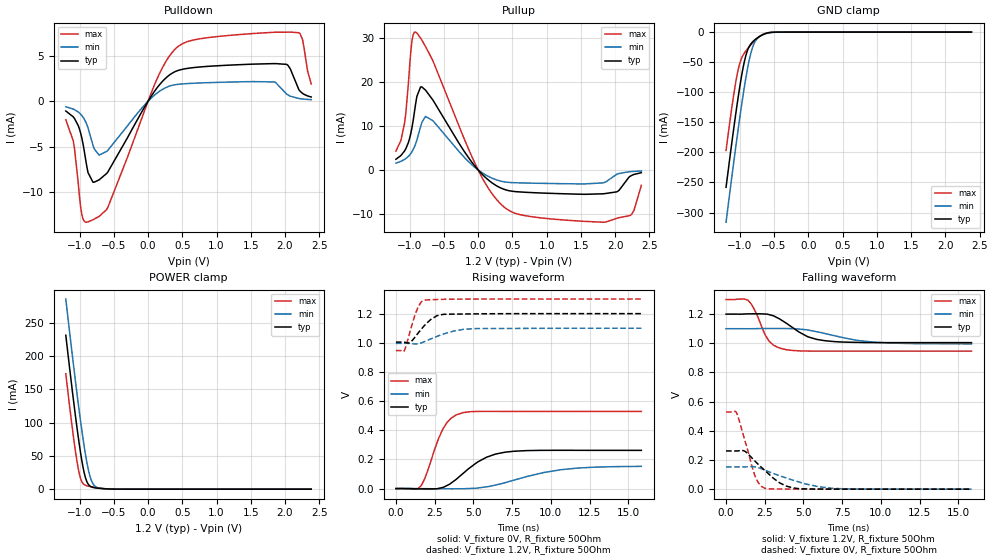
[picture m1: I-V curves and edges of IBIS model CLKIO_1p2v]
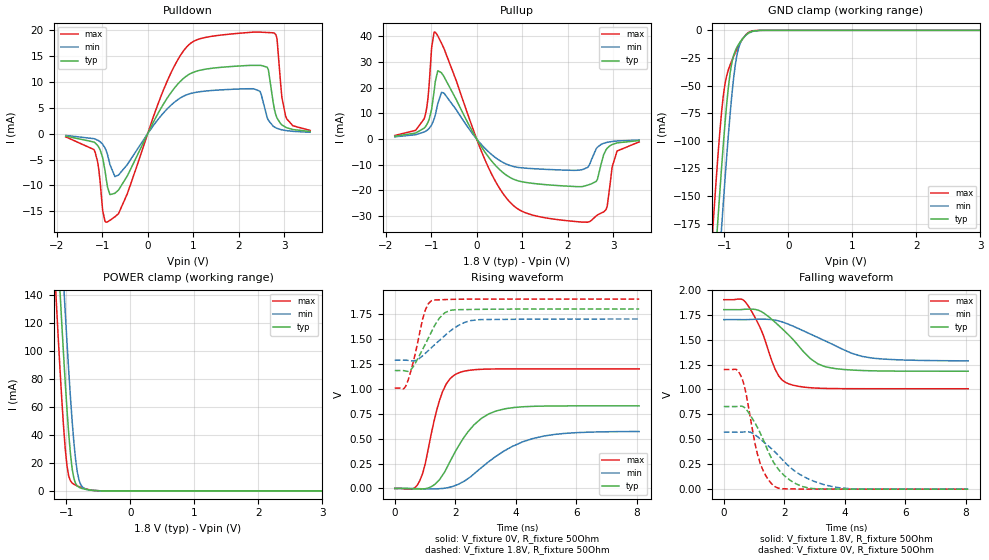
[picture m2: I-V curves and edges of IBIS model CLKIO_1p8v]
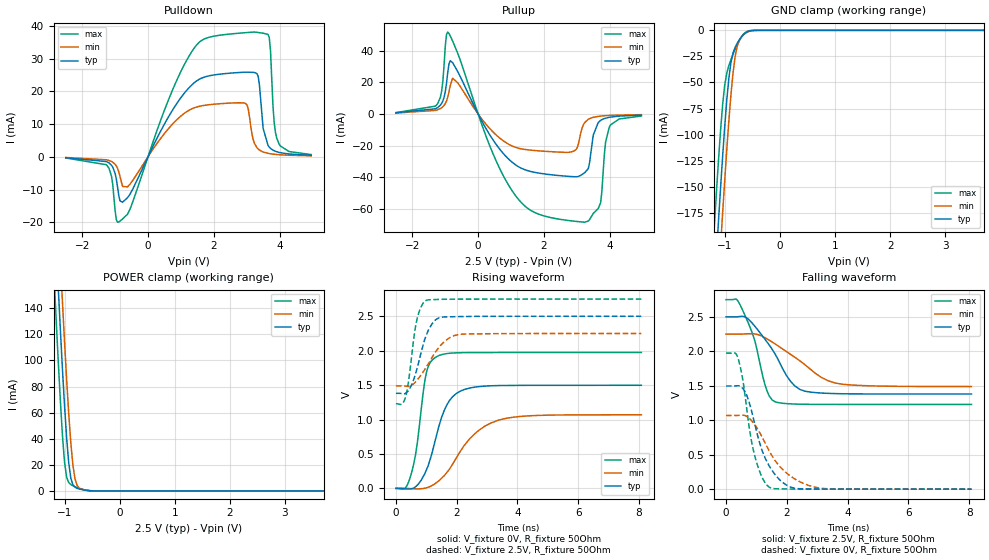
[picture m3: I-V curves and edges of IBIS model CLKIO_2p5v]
|Texas Instruments Incorporated
|Low power Stereo ADC with Embeded miniDSP
|for Wireless Handsets and Portable Audio
| Marketing part#   Voltage Range(Digital)   Package-type   #pin
|TLV320ADC3101IRGER   1.2V to 3.3V   VQFN   24
|TLV320ADC3101IRGET   1.2V to 3.3V   VQFN   24
[IBIS Ver]   4.0
[File name]   tlv320adc3101.ibs
[File Rev]   1.0
[Date]   06/13/2011
[Source]   Texas Instruments Incorporated.
   Analog-eLab, HPA
   12500 TI Blvd
   Dallas, TX -75243
   For Support e-mail: elab_ibis@list.ti.com
[Notes]   Revision History:
   1.0: 06/13/2011
   - Initial version of the model
   - Initial Model generated from simulations.
   - Model not matched to measurements
   - ccomp values are based on PVT conditions although listed
   in numerical order.
   - CLK_IO model is split into 4 models (CLKIO_1p2v, CLKIO_1p8v
   CLKIO_2p5v, CLKIO_3p3v) based operating voltages (1.2V, 1.8V,
   2.5V and 3.3V).
   - DATA model is split into 4 models (DATA_1p2v, DATA_1p8v
   DATA_2p5v, DATA_3p3v) based operating voltages (1.2V, 1.8V,
   2.5V and 3.3V).
   - INPUT model is split into 4 models (INPUT_1p2v, INPUT_1p8v
   INPUT_2p5v, INPUT_3p3v) based operating voltages (1.2V, 1.8V,
   2.5V and 3.3V).
   - I2C_IO model is split into 4 models (SDA_1p2v, SDA_1p8v
   SDA_2p5v, SDA_3p3v) based operating voltages (1.2V, 1.8V,
   2.5V and 3.3V).
   - Non-monotonicity warnings on DATA and CLK_IO buffer are
   reflection of spice simulations and can be ignored.
[Disclaimer]
 This product is designed as an aid for customers of Texas Instruments.
 No warranties, either expressed or implied, with respect to this third
 party software (if any) or with respect to its fitness for any
 particular purpose is claimed by Texas Instruments or the author. The
 software (if any) is provided solely on an "as is" basis. The entire
 risk as to its quality and performance is with the customer
[Copyright] (C) Copyright 2011 Texas Instruments Incorporated.
   All rights reserved.
|   TLV320ADC3101
[Component]   tlv320adc3101
[Manufacturer] TI
[Package]   | 24 pin  package
| variable   typ   min   max
R_pkg   0.0746   0.0381   0.0838
L_pkg   1.09nH   0.81nH   1.21nH
C_pkg   0.148pF   0.126pF   0.195pF
|-------------------------PIN------------------------------------------------
[Pin] signal_name  model_name  R_pin  L_pin C_pin
1   BCLK   CLK_IO   0.07924   1.11525nH   0.12716pF
2   WCLK   CLK_IO   0.07327   1.05316nH   0.1487pF
3   DOUT   DATA   0.07354   1.05587nH   0.14822pF
4   RESETB   INPUT   0.07981   1.14793nH   0.1523pF
5   MICBIAS1   TERM   0.07489   1.07511nH   0.14724pF
6   IN3L   TERM   0.07839   1.12703nH   0.15083pF
7   IN2L   TERM   0.08148   1.17211nH   0.15382pF
8   IN1L   TERM   0.07748   1.11307nH   0.15103pF
9   AVSS   GND   0.03814   0.80558nH   0.15549pF
10   AVDD   POWER   0.07565   1.08748nH   0.12622pF
11   IN1R   TERM   0.07727   1.10694nH   0.15pF
12   IN2R   TERM   0.08077   1.1574nH   0.15299pF
13   IN3R   TERM   0.07839   1.11986nH   0.15072pF
14   MICBIAS2   TERM   0.07489   1.06758nH   0.14704pF
15   I2C_ADR0   INPUT   0.07998   1.14372nH   0.15228pF
16   I2C_ADR1   INPUT   0.07361   1.04912nH   0.14805pF
17   SCL   I2C_IO   0.07322   1.04451nH   0.14849pF
18   SDA   I2C_IO   0.07924   1.13822nH   0.12709pF
19   DMDIN_GPIO1   CLK_IO   0.08359   1.20475nH   0.13135pF
20   DMCLK_GPIO2   CLK_IO   0.07633   1.09324nH   0.1509pF
21   IVODD   POWER   0.07496   1.07238nH   0.15063pF
22   DVDD   POWER   0.07812   1.12112nH   0.15804pF
23   DVSS   GND   0.04448   0.97782nH   0.19585pF
24   MCLK   INPUT   0.08381   1.20712nH   0.15521pF
[Model Selector] CLK_IO
CLKIO_3p3v  3.3V cmos I/O
CLKIO_2p5v  2.5V cmos I/O
CLKIO_1p8v  1.8V cmos I/O
CLKIO_1p2v  1.2V cmos I/O
[Model Selector] DATA
DATA_3p3v   3.3V tristate output
DATA_2p5v   2.5V tristate output
DATA_1p8v   1.8V tristate output
DATA_1p2v   1.2V tristate output
[Model Selector] INPUT
INPUT_3p3v  3.3V cmos input
INPUT_2p5v  2.5V cmos input
INPUT_1p8v  1.8V cmos input
INPUT_1p2v  1.2V cmos input
[Model Selector] I2C_IO
SDA_3p3v  3.3V open I/O
SDA_2p5v  2.5V open I/O
SDA_1p8v  1.8V open I/O
SDA_1p2v  1.2V open I/O
[Model]  TERM
Model_type Terminator
C_comp   0   0   0
[Voltage Range]  3.3  3.0  3.6
[Temperature Range] 27   85   -40
| Models and submodels in the file (17): CLKIO_1p2v (I/O), CLKIO_1p8v (I/O), CLKIO_2p5v (I/O), CLKIO_3p3v (I/O), DATA_1p2v (3-state), DATA_1p8v (3-state), DATA_2p5v (3-state), DATA_3p3v (3-state), INPUT_1p2v (Input), INPUT_1p8v (Input), INPUT_2p5v (Input), INPUT_3p3v (Input), SDA_1p2v (I/O_open_drain), SDA_1p8v (I/O_open_drain), SDA_2p5v (I/O_open_drain), SDA_3p3v (I/O_open_drain), TERM (Terminator)
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|   CLKIO_1p2v
[Model]   CLKIO_1p2v
Model_type   I/O
Polarity   Non-Inverting
Enable   Active-High
Vinl = 0.36
Vinh = 0.84
Vmeas = 0.6
Vref = 0
Cref = 5pF
Rref = 1000000
|   typ   min   max
C_comp   1.630pF   1.592pF   1.693pF
[Voltage Range]   1.2   1.1   1.3
[Temperature Range]   27   85   -40
[Pullup Reference]   1.2   1.1   1.3
[Pulldown Reference]   -0   -0   -0
[Power Clamp Reference]   1.2   1.1   1.3
[GND Clamp Reference]   -0   -0   -0
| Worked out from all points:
|   slope of the pulldown table from 0 to 0.18 V, typ, clamps not added: 93.3 ohm
|   slope of the pullup table from 0 to 0.18 V, typ, clamps not added: 67.6 ohm
|   GND clamp passes 1 mA (typ) near -0.57 V on its own axis
|   POWER clamp passes 1 mA (typ) near -0.68 V on its own axis
|   falling waveform, V_fixture 1.2V, R_fixture 50Ohm: 20-80 % time 1.76ns typ, 2.87ns min, 919ps max; typ from 1.2 V to 1 V
|   rising waveform, V_fixture 0V, R_fixture 50Ohm: 20-80 % time 2ns typ, 3.54ns min, 1.13ns max; typ from 0 V to 0.262 V
|   rising waveform, V_fixture 1.2V, R_fixture 50Ohm: 20-80 % time 996ps typ, 1.64ns min, 610ps max; typ from 1 V to 1.2 V
|   falling waveform, V_fixture 0V, R_fixture 50Ohm: 20-80 % time 1.64ns typ, 2.66ns min, 845ps max; typ from 0.262 V to 0 V
[Pulldown]
|   Voltage   I(typ)   I(min)   I(max)
-1.2V     -1.07mA    -597.3uA   -2.042mA
-1.092V   -1.709mA   -856.2uA   -4.33mA
-1.02V    -2.651mA   -1.171mA   -8.868mA
-966mV    -4.044mA   -1.567mA   -12.48mA
-894mV    -7.151mA   -2.544mA   -13.31mA
-714mV    -8.651mA   -5.923mA   -12.68mA
-588mV    -7.806mA   -5.41mA    -11.71mA
168mV     1.822mA    1.102mA    3.055mA
492mV     3.504mA    1.906mA    6.299mA
2.022V    4.065mA    805.4uA    7.611mA
2.202V    1.268mA    305.9uA    7.546mA
2.382V    470.8uA    178.6uA    1.904mA
[GND Clamp]
|   Voltage   I(typ)   I(min)   I(max)
-1.2V     -258.1mA   -316.1mA   -196.8mA
-1.11V    -179mA     -235.8mA   -121mA
-1.038V   -119.8mA   -174mA     -70.54mA
-984mV    -79.98mA   -130mA     -46.43mA
-930mV    -47.68mA   -89.38mA   -34.41mA
-876mV    -27.29mA   -54.35mA   -26.35mA
-822mV    -17.42mA   -28.48mA   -19.29mA
-768mV    -11.74mA   -14.04mA   -12.97mA
-714mV    -7.456mA   -7.504mA   -7.628mA
-624mV    -2.511mA   -2.629mA   -1.885mA
-534mV    -448.7uA   -620uA     -192.6uA
2.382V    0A         0A         0A
[Pullup]
|   Voltage   I(typ)   I(min)   I(max)
-1.2V     2.421mA    1.547mA    4.272mA
-1.074V   4.296mA    2.378mA    10.6mA
-966mV    9.578mA    4.11mA     29.26mA
-912mV    15.02mA    5.927mA    31.26mA
-840mV    18.83mA    9.821mA    29.89mA
-768mV    18.09mA    12.13mA    27.99mA
6mV       -105.3uA   -68.85uA   -187.8uA
420mV     -4.595mA   -2.784mA   -8.894mA
1.86V     -5.348mA   -2.744mA   -11.81mA
2.04V     -4.823mA   -895.3uA   -10.89mA
2.238V    -1.262mA   -368.8uA   -10.11mA
2.382V    -626.9uA   -250.3uA   -3.496mA
[POWER Clamp]
|   Voltage   I(typ)   I(min)   I(max)
-1.2V     231.1mA    285.3mA    173.2mA
-1.128V   167.6mA    221.3mA    110.7mA
-1.074V   122.1mA    174.7mA    67.66mA
-1.038V   93.31mA    144.7mA    42.54mA
-1.002V   66.55mA    115.7mA    22.83mA
-948mV    32.67mA    75.35mA    8.401mA
-894mV    11.57mA    41.03mA    5.093mA
-840mV    4.122mA    16.94mA    3.804mA
-804mV    2.641mA    8.113mA    3.132mA
-768mV    1.932mA    3.889mA    2.523mA
-480mV    49.56uA    80.74uA    34.71uA
2.382V    0A         0A         0A
[Ramp]
R_load = 50
|   typ   min   max
dV/dt_r   0.157257/2.00205e-009 0.0913656/3.53688e-009  0.317475/1.12719e-009
dV/dt_f   0.117245/1.76151e-009  0.062354/2.86788e-009  0.212217/9.19327e-010
[Falling Waveform]
V_fixture = 1.2V
V_fixture_min = 1.1V
V_fixture_max = 1.3V
R_fixture = 50Ohm
C_fixture = 0F
|   Time   V(typ)   V(min)   V(max)
0s        1.2V       1.1V       1.3V
1.423ns   1.202V     1.1V       1.295V
1.857ns   1.202V     1.1V       1.226V
2.507ns   1.201V     1.101V     1.061V
2.772ns   1.197V     1.101V     1.015V
3.906ns   1.136V     1.101V     955.9mV
5.271ns   1.045V     1.091V     946.7mV
6.438ns   1.017V     1.066V     946.2mV
9.582ns   1.005V     1.007V     946.3mV
15.84ns   1.005V     996.1mV    946.3mV
[Rising Waveform]
V_fixture = 0V
V_fixture_min = 0V
V_fixture_max = 0V
R_fixture = 50Ohm
C_fixture = 0F
|   Time   V(typ)   V(min)   V(max)
0s        -1.318uV   -3.119uV   -2.104uV
1.207ns   -1.529mV   132.3uV    -4.123mV
1.64ns    -2.22mV    -319uV     21.2mV
3.037ns   7.794mV    -1.349mV   409.6mV
3.567ns   37.87mV    -1.431mV   483.3mV
4.362ns   106.2mV    -1.186mV   521.5mV
5.855ns   215.3mV    12mV       529.7mV
7.021ns   249.2mV    39.65mV    529.4mV
10.66ns   262.5mV    129.4mV    529.1mV
15.84ns   262.1mV    152.3mV    529.1mV
[Rising Waveform]
V_fixture = 1.2V
V_fixture_min = 1.1V
V_fixture_max = 1.3V
R_fixture = 50Ohm
C_fixture = 0F
|   Time   V(typ)   V(min)   V(max)
0s        1.005V     996.1mV    946.3mV
533.2ps   1.004V     996.5mV    945.1mV
942ps     1.005V     995mV      1.088V
1.423ns   1.065V     993.2mV    1.245V
1.64ns    1.094V     999.4mV    1.282V
1.857ns   1.12V      1.008V     1.293V
2.653ns   1.186V     1.044V     1.297V
3.06ns    1.195V     1.06V      1.298V
5.179ns   1.198V     1.098V     1.3V
15.84ns   1.2V       1.1V       1.3V
[Falling Waveform]
|Gnd
V_fixture = 0V
V_fixture_min = 0V
V_fixture_max = 0V
R_fixture = 50Ohm
C_fixture = 0F
|   Time   V(typ)   V(min)   V(max)
0s        262.1mV    152.5mV    529.1mV
682.4ps   262mV      152.3mV    522.6mV
1.169ns   262.3mV    152.6mV    351.2mV
1.857ns   193.5mV    153mV      93.19mV
2.074ns   170.8mV    147.7mV    45.25mV
2.507ns   128.1mV    130.5mV    5.84mV
3.467ns   42.82mV    91.7mV     1.137mV
4.688ns   3.395mV    49.91mV    156.3uV
7.671ns   291.7uV    1.874mV    2.37uV
15.84ns   -1.062uV   18.06uV    128.5nV
|   CLKIO_1p8v
[Model]   CLKIO_1p8v
Model_type   I/O
Polarity   Non-Inverting
Enable   Active-High
Vinl = 0.54
Vinh = 1.26
Vmeas = 0.9
Vref = 0
Cref = 5pF
Rref = 1000000
|   typ   min   max
C_comp   1.630pF   1.592pF   1.693pF
[Voltage Range]   1.8   1.7   1.9
[Temperature Range]   27   85   -40
[Pullup Reference]   1.8   1.7   1.9
[Pulldown Reference]   -0   -0   -0
[Power Clamp Reference]   1.8   1.7   1.9
[GND Clamp Reference]   -0   -0   -0
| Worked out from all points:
|   slope of the pulldown table from 0 to 0.27 V, typ, clamps not added: 59 ohm
|   slope of the pullup table from 0 to 0.27 V, typ, clamps not added: 37.3 ohm
|   GND clamp passes 1 mA (typ) near -0.57 V on its own axis
|   POWER clamp passes 1 mA (typ) near -0.68 V on its own axis
|   falling waveform, V_fixture 1.8V, R_fixture 50Ohm: 20-80 % time 1.19ns typ, 1.76ns min, 694ps max; typ from 1.8 V to 1.18 V
|   rising waveform, V_fixture 0V, R_fixture 50Ohm: 20-80 % time 1.06ns typ, 1.65ns min, 567ps max; typ from 0 V to 0.828 V
|   rising waveform, V_fixture 1.8V, R_fixture 50Ohm: 20-80 % time 639ps typ, 949ps min, 403ps max; typ from 1.18 V to 1.8 V
|   falling waveform, V_fixture 0V, R_fixture 50Ohm: 20-80 % time 870ps typ, 1.33ns min, 495ps max; typ from 0.828 V to 0 V
[Pulldown]
|   Voltage   I(typ)   I(min)   I(max)
-1.8V     -446.7uA   -316.8uA   -599.3uA
-1.179V   -1.6mA     -947.7uA   -3.058mA
-1.071V   -2.646mA   -1.378mA   -7.075mA
-990mV    -4.574mA   -2.008mA   -14.74mA
-882mV    -10.33mA   -4.037mA   -17.03mA
-639mV    -10.88mA   -7.975mA   -15.44mA
819mV     10.93mA    7.395mA    16.38mA
2.331V    13.24mA    8.707mA    19.67mA
2.655V    12.35mA    2.589mA    19.58mA
2.817V    3.697mA    1.159mA    19.19mA
3.033V    1.263mA    634.3uA    3.405mA
3.573V    443.3uA    289.3uA    650.2uA
[GND Clamp]
|   Voltage   I(typ)   I(min)   I(max)
-1.8V     -825.7mA   -883.1mA   -764.8mA
-1.179V   -239.3mA   -297.1mA   -178.4mA
-1.125V   -191.9mA   -248.9mA   -133mA
-1.098V   -168.8mA   -225.3mA   -111.7mA
-1.044V   -124.5mA   -179mA     -74.1mA
-990mV    -84.11mA   -134.8mA   -48.37mA
-936mV    -50.74mA   -93.67mA   -35.44mA
-882mV    -28.93mA   -57.86mA   -27.19mA
-828mV    -18.22mA   -30.79mA   -20.04mA
-747mV    -9.958mA   -10.88mA   -10.76mA
-612mV    -2.077mA   -2.232mA   -1.464mA
3.573V    0A         0A         0A
[Pullup]
|   Voltage   I(typ)   I(min)   I(max)
-1.8V     1.07mA     844.6uA    1.357mA
-1.152V   4.258mA    2.717mA    7.917mA
-1.071V   6.428mA    3.67mA     15.74mA
-936mV    18.47mA    7.689mA    41.63mA
-855mV    26.58mA    13.72mA    40.19mA
-720mV    24.34mA    17.91mA    35.31mA
252mV     -6.828mA   -4.846mA   -10.85mA
954mV     -16.5mA    -11.17mA   -27.75mA
2.493V    -17.65mA   -9.494mA   -32.08mA
2.844V    -4.206mA   -1.404mA   -27.53mA
3.087V    -1.515mA   -777.6uA   -4.683mA
3.573V    -628uA     -402.2uA   -1.128mA
[POWER Clamp]
|   Voltage   I(typ)   I(min)   I(max)
-1.8V     798.6mA    851.4mA    743.1mA
-1.179V   212.3mA    266.5mA    154.6mA
-1.152V   188.5mA    242.4mA    131.1mA
-1.098V   142mA      195.2mA    86.23mA
-1.044V   97.98mA    149.6mA    46.43mA
-1.017V   77.4mA     127.6mA    30.18mA
-990mV    58.24mA    106.4mA    18mA
-909mV    15.86mA    49.74mA    5.628mA
-855mV    5.278mA    22.34mA    4.111mA
-801mV    2.564mA    7.615mA    3.079mA
-450mV    23.52uA    44.09uA    13.85uA
3.573V    0A         0A         0A
[Ramp]
R_load = 50
|   typ   min   max
dV/dt_r   0.497073/1.06086e-009  0.342582/1.65226e-009  0.719771/5.67278e-010
dV/dt_f   0.370361/1.18967e-009  0.247646/1.75578e-009  0.535854/6.94284e-010
[Falling Waveform]
V_fixture = 1.8V
V_fixture_min = 1.7V
V_fixture_max = 1.9V
R_fixture = 50Ohm
C_fixture = 0F
|   Time   V(typ)   V(min)   V(max)
0s        1.8V       1.7V       1.9V
753.7ps   1.804V     1.7V       1.861V
1.204ns   1.786V     1.704V     1.618V
1.697ns   1.673V     1.695V     1.202V
1.932ns   1.607V     1.677V     1.092V
2.167ns   1.538V     1.65V      1.054V
2.859ns   1.309V     1.556V     1.017V
3.349ns   1.228V     1.487V     1.01V
4.909ns   1.187V     1.314V     1.007V
8.073ns   1.183V     1.287V     1.007V
[Rising Waveform]
V_fixture = 0V
V_fixture_min = 0V
V_fixture_max = 0V
R_fixture = 50Ohm
C_fixture = 0F
|   Time   V(typ)   V(min)   V(max)
0s        -6.278uV   -2.564uV   -11.23uV
606.8ps   -4.343mV   -81.27uV   -2.123mV
828.1ps   -5.588mV   -2.675mV   78.44mV
1.485ns   91.64mV    -2.191mV   890.4mV
1.697ns   194.1mV    5.008mV    1.046V
2.05ns    396.1mV    35.81mV    1.152V
2.859ns   702.6mV    208.3mV    1.195V
3.651ns   799.9mV    382.7mV    1.199V
5.256ns   827.4mV    541.2mV    1.199V
8.073ns   828.4mV    571mV      1.2V
[Rising Waveform]
V_fixture = 1.8V
V_fixture_min = 1.7V
V_fixture_max = 1.9V
R_fixture = 50Ohm
C_fixture = 0F
|   Time   V(typ)   V(min)   V(max)
0s        1.183V     1.286V     1.007V
289.8ps   1.182V     1.287V     1.001V
389ps     1.176V     1.286V     1.044V
606.8ps   1.222V     1.279V     1.264V
922ps     1.397V     1.332V     1.702V
1.016ns   1.452V     1.358V     1.795V
1.204ns   1.566V     1.41V      1.882V
1.648ns   1.762V     1.532V     1.895V
2.512ns   1.795V     1.684V     1.899V
8.073ns   1.8V       1.7V       1.9V
[Falling Waveform]
|Gnd
V_fixture = 0V
V_fixture_min = 0V
V_fixture_max = 0V
R_fixture = 50Ohm
C_fixture = 0F
|   Time   V(typ)   V(min)   V(max)
0s        828.4mV    571.6mV    1.2V
400ps     828.4mV    571.4mV    1.201V
557.9ps   832.5mV    571.7mV    1.14V
704.7ps   812.2mV    574.4mV    1.001V
1.016ns   671.7mV    548.8mV    478.4mV
1.204ns   562.1mV    503.7mV    258.2mV
1.697ns   246mV      370.7mV    24.38mV
2.416ns   49.46mV    167.2mV    1.866mV
3.596ns   1.62mV     24.72mV    171uV
8.073ns   1.935uV    79.25uV    -2.062uV
|   CLKIO_2p5v
[Model]   CLKIO_2p5v
Model_type   I/O
Polarity   Non-Inverting
Enable   Active-High
Vinl = 0.75
Vinh = 1.75
Vmeas = 1.25
Vref = 0
Cref = 5pF
Rref = 1000000
|   typ   min   max
C_comp   1.630pF   1.592pF   1.693pF
[Voltage Range]   2.5   2.25   2.75
[Temperature Range]   27   85   -40
[Pullup Reference]   2.5   2.25   2.75
[Pulldown Reference]   -0   -0   -0
[Power Clamp Reference]   2.5   2.25   2.75
[GND Clamp Reference]   -0   -0   -0
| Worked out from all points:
|   slope of the pulldown table from 0 to 0.375 V, typ, clamps not added: 48.9 ohm
|   slope of the pullup table from 0 to 0.375 V, typ, clamps not added: 27 ohm
|   GND clamp passes 1 mA (typ) near -0.57 V on its own axis
|   POWER clamp passes 1 mA (typ) near -0.68 V on its own axis
|   falling waveform, V_fixture 2.5V, R_fixture 50Ohm: 20-80 % time 953ps typ, 1.42ns min, 572ps max; typ from 2.5 V to 1.38 V
|   rising waveform, V_fixture 0V, R_fixture 50Ohm: 20-80 % time 628ps typ, 1.12ns min, 354ps max; typ from 0 V to 1.5 V
|   rising waveform, V_fixture 2.5V, R_fixture 50Ohm: 20-80 % time 444ps typ, 700ps min, 282ps max; typ from 1.38 V to 2.5 V
|   falling waveform, V_fixture 0V, R_fixture 50Ohm: 20-80 % time 673ps typ, 986ps min, 449ps max; typ from 1.5 V to 0 V
[Pulldown]
|   Voltage   I(typ)   I(min)   I(max)
-2.5V     -290.5uA   -214.9uA   -365.9uA
-1.262V   -1.448mA   -911.1uA   -2.421mA
-887.5mV  -11.93mA   -4.616mA   -19.88mA
-625mV    -12.51mA   -9.182mA   -17.54mA
1.4V      22.56mA    14.92mA    33.12mA
2.975V    25.83mA    16.23mA    37.89mA
3.237V    25.73mA    4.081mA    38.06mA
3.35V     24.52mA    2.367mA    37.94mA
3.688V    2.949mA    982uA      36.34mA
3.837V    1.849mA    772.8uA    10.3mA
3.987V    1.335mA    635.9uA    3.857mA
4.963V    465.7uA    292.8uA    680.3uA
[GND Clamp]
|   Voltage   I(typ)   I(min)   I(max)
-2.5V     -1.51A     -1.565A    -1.451A
-1.188V   -246.9mA   -304.8mA   -185.8mA
-1.113V   -181.2mA   -237.9mA   -123mA
-1.075V   -149.6mA   -205.4mA   -94.66mA
-1.038V   -119.4mA   -173.6mA   -70.25mA
-1V       -91.19mA   -142.8mA   -52mA
-925mV    -45.24mA   -85.86mA   -33.59mA
-887.5mV  -30.55mA   -61.18mA   -27.96mA
-812.5mV  -16.25mA   -25.13mA   -18.12mA
-775mV    -12.38mA   -15.34mA   -13.74mA
-587.5mV  -1.357mA   -1.556mA   -829.3uA
4.963V    0A         0A         0A
[Pullup]
|   Voltage   I(typ)   I(min)   I(max)
-2.5V     744.4uA    601.2uA    890.3uA
-1.225V   4.149mA    2.755mA    6.802mA
-1.113V   6.631mA    3.932mA    14.12mA
-925mV    26.14mA    10.57mA    51.83mA
-775mV    32.49mA    22.62mA    46.15mA
1.1V      -31.59mA   -20.81mA   -50.59mA
2.9V      -39.66mA   -23.53mA   -67.78mA
3.237V    -37.23mA   -5.486mA   -68.46mA
3.725V    -4.042mA   -1.335mA   -56.09mA
3.875V    -2.647mA   -1.07mA    -17.83mA
3.987V    -2.09mA    -929.5uA   -8.29mA
4.963V    -725uA     -431.6uA   -1.274mA
[POWER Clamp]
|   Voltage   I(typ)   I(min)   I(max)
-2.5V     1.482A     1.533A     1.43A
-1.188V   219.9mA    274.1mA    162.1mA
-1.15V    186.7mA    240.7mA    129.4mA
-1.113V   154.3mA    207.8mA    97.93mA
-1.075V   122.9mA    175.6mA    68.41mA
-1.038V   92.92mA    144.2mA    42.22mA
-1V       65.14mA    114.1mA    21.96mA
-925mV    21.79mA    59.79mA    6.423mA
-850mV    4.839mA    20.42mA    4.006mA
-775mV    2.042mA    4.456mA    2.637mA
-437.5mV  16.91uA    33.64uA    9.233uA
4.963V    0A         0A         0A
[Ramp]
R_load = 50
|   typ   min   max
dV/dt_r   0.898621/6.2751e-010   0.64165/1.12369e-009   1.1843/3.53629e-010
dV/dt_f   0.671694/9.53036e-010  0.456503/1.42453e-009  0.912502/5.72135e-010
[Falling Waveform]
V_fixture = 2.5V
V_fixture_min = 2.25V
V_fixture_max = 2.75V
R_fixture = 50Ohm
C_fixture = 0F
|   Time   V(typ)   V(min)   V(max)
0s        2.5V       2.25V      2.75V
323.8ps   2.5V       2.25V      2.758V
470.4ps   2.506V     2.25V      2.667V
892.5ps   2.393V     2.255V     2.229V
1.346ns   2.136V     2.181V     1.427V
1.615ns   1.96V      2.107V     1.268V
2.124ns   1.564V     1.956V     1.238V
2.591ns   1.422V     1.808V     1.232V
3.858ns   1.385V     1.521V     1.23V
8.076ns   1.381V     1.489V     1.229V
[Rising Waveform]
V_fixture = 0V
V_fixture_min = 0V
V_fixture_max = 0V
R_fixture = 50Ohm
C_fixture = 0F
|   Time   V(typ)   V(min)   V(max)
0s        12.06uV    -14.35uV   357.3uV
470.4ps   -7.962mV   -3.206mV   161mV
641.9ps   21.96mV    -6.089mV   479.6mV
1.018ns   284.6mV    10.01mV    1.71V
1.346ns   788.1mV    88.11mV    1.915V
1.668ns   1.206V     227.3mV    1.957V
1.99ns    1.379V     444mV      1.968V
2.566ns   1.469V     782.4mV    1.973V
3.372ns   1.493V     990mV      1.974V
8.076ns   1.498V     1.069V     1.974V
[Rising Waveform]
V_fixture = 2.5V
V_fixture_min = 2.25V
V_fixture_max = 2.75V
R_fixture = 50Ohm
C_fixture = 0F
|   Time   V(typ)   V(min)   V(max)
0s        1.381V     1.489V     1.23V
186.7ps   1.378V     1.489V     1.224V
308.6ps   1.378V     1.486V     1.317V
400ps     1.415V     1.482V     1.513V
512.8ps   1.501V     1.496V     1.903V
704.6ps   1.758V     1.578V     2.479V
1.018ns   2.244V     1.775V     2.735V
1.418ns   2.479V     2.052V     2.745V
2.079ns   2.495V     2.236V     2.749V
8.076ns   2.5V       2.25V      2.75V
[Falling Waveform]
|Gnd
V_fixture = 0V
V_fixture_min = 0V
V_fixture_max = 0V
R_fixture = 50Ohm
C_fixture = 0F
|   Time   V(typ)   V(min)   V(max)
0s        1.498V     1.069V     1.974V
400ps     1.501V     1.07V      1.891V
516.6ps   1.477V     1.073V     1.674V
638.3ps   1.403V     1.066V     1.315V
892.5ps   1.04V      965.5mV    577.6mV
1.143ns   619.8mV    792.5mV    214.9mV
1.424ns   334.1mV    550.3mV    27.43mV
1.99ns    58.78mV    235.1mV    3.284mV
2.928ns   2.395mV    28.21mV    701.6uV
8.076ns   -2.571uV   25.18uV    -8.221uV
